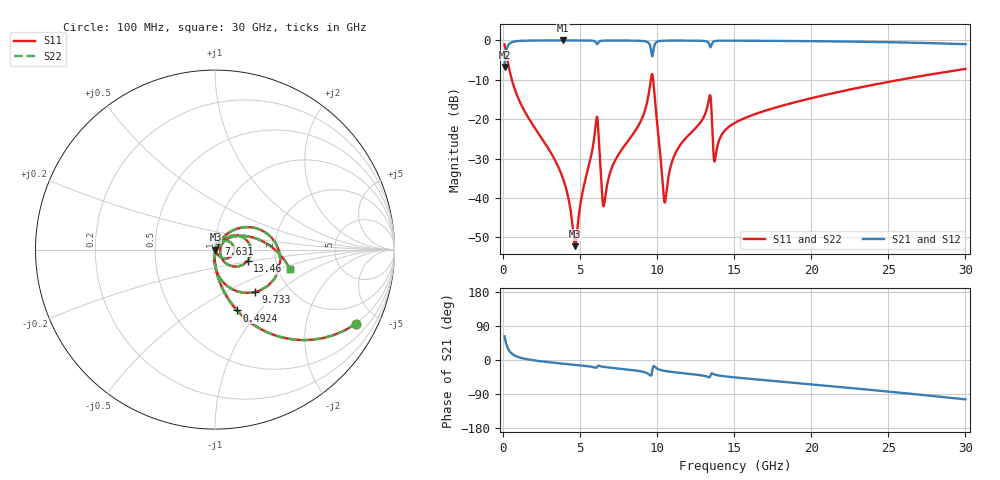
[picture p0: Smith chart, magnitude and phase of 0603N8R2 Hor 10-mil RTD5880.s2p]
# GHz S MA R 50
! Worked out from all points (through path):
!   3201 points, 100 MHz to 30 GHz, reference 50 ohm
!   highest |S21| = -0.02 dB at 3.894 GHz (marker M1); lowest = -6.7 dB at 100 MHz (marker M2)
!   group delay of S21, straight-line fit = 10.2 ps
!   lowest |S11| = -52.3 dB at 4.678 GHz (marker M3), VSWR 1.00, Z = 50.2 - j0.0575 ohm
!   |S11| at or under -10 dB: 569.3 MHz to 9.586 GHz (9.017 GHz wide, 178 % of centre); 9.741 GHz to 25.76 GHz (16.02 GHz wide, 90.3 % of centre)
!   |S22| runs from -52.3 to -1.0 dB; largest |S21 - S12| = 0
!   S11 on the Smith chart (normalised r, x): 100 MHz: 0.98, -3.81; 492.4 MHz: 0.98, -0.77; 7.631 GHz: 1.04, +0.07; 9.733 GHz: 1.36, -0.72; 13.46 GHz: 1.43, -0.19; 30 GHz: 2.32, -0.63
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0.1  0.8871 -27.8  0.4614 62.2  0.4614 62.2  0.8871 -27.8
0.4924375  0.3606 -70.1  0.9321 19.8  0.9321 19.8  0.3606 -70.1
3.893562  0.01748 -93.0  0.9977 -9.8  0.9977 -9.8  0.01748 -93.0
4.678438  0.002438 -13.6  0.9975 -12.9  0.9975 -12.9  0.002438 -13.6
5.089563  0.01009 58.9  0.997 -14.6  0.997 -14.6  0.01009 58.9
6.042625  0.09548 24.6  0.9303 -20.5  0.9303 -20.5  0.09548 24.6
6.173438  0.0755 -41.6  0.9318 -15.1  0.9318 -15.1  0.0755 -41.6
6.407031  0.01289 -48.0  0.9888 -17.3  0.9888 -17.3  0.01289 -48.0
6.547187  0.008056 12.2  0.993 -18.3  0.993 -18.3  0.008056 12.2
7.631062  0.0392 61.1  0.9952 -23.2  0.9952 -23.2  0.0392 61.1
8.892469  0.09077 55.1  0.9874 -29.6  0.9874 -29.6  0.09077 55.1
9.425062  0.1954 39.1  0.934 -36.8  0.934 -36.8  0.1954 39.1
9.733406  0.3261 -46.5  0.7017 -17.6  0.7017 -17.6  0.3261 -46.5
10.06978  0.06421 -91.4  0.9733 -24.2  0.9733 -24.2  0.06421 -91.4
10.51828  0.008992 -6.0  0.9916 -29.0  0.9916 -29.0  0.008992 -6.0
11.24709  0.03908 49.6  0.9941 -33.0  0.9941 -33.0  0.03908 49.6
13.46156  0.1922 -19.5  0.818 -40.6  0.818 -40.6  0.1922 -19.5
13.76991  0.03191 16.2  0.9812 -38.9  0.9812 -38.9  0.03191 16.2
15.05  0.08984 41.1  0.9911 -46.0  0.9911 -46.0  0.08984 41.1
20.03956  0.1853 24.1  0.9775 -64.4  0.9775 -64.4  0.1853 24.1
25.01978  0.2973 5.5  0.9486 -83.4  0.9486 -83.4  0.2973 5.5
30  0.4335 -14.7  0.8939 -103.8  0.8939 -103.8  0.4335 -14.7
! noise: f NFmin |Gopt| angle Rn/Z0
0.1  0.0003247  0.9267  0.5979  0.0009821
3.417  0.003743  0.7966  9.479  0.00378
6.743  0.008546  0.8224  18.54  0.009838
10.06  0.02389  0.9018  27.57  0.05025
13.39  0.0577  0.9451  36.42  0.2126
16.7  0.01268  0.7265  44.77  0.007912
20.03  0.01461  0.7198  53.08  0.008315
23.35  0.01678  0.7194  61.16  0.008858
26.67  0.01914  0.7223  69.03  0.009394
30  0.02172  0.7277  76.7  0.009909
